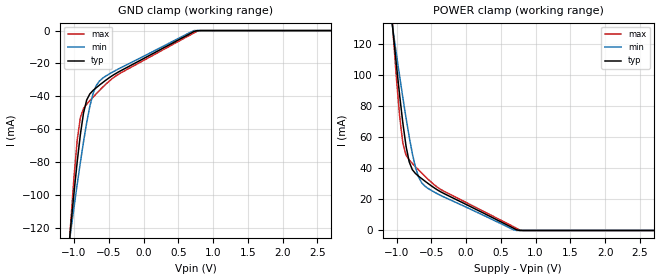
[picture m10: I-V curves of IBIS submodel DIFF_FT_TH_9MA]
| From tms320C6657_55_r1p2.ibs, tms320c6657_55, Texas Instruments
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|   Model Cell DIFF_FT_TH_9MA
|DIFF_FT_TH_9MA
[Submodel]   DIFF_FT_TH_9MA
Submodel_type   Dynamic_clamp
[POWER_clamp]
|   voltage   I(typ)   I(min)   I(max)
-1.5V     344.8mA    277.3mA    440.9mA
-1.091V   146.5mA    141.4mA    153.5mA
-1.046V   125.7mA    127mA      124.3mA
-954.6mV  86.42mA    98.78mA    72.95mA
-909.2mV  68.87mA    85.24mA    56mA
-863.7mV  54.18mA    72.3mA     48.37mA
-818.2mV  44.11mA    60.2mA     45.3mA
-727.3mV  36.59mA    40.46mA    40.96mA
-636.4mV  33.23mA    30.51mA    36.83mA
-545.5mV  30.15mA    26.97mA    32.86mA
772.8mV   0A         0A         343.5uA
3V        0A         0A         0A
[GND_clamp]
|   voltage   I(typ)   I(min)   I(max)
-1.5V     -337.5mA   -271.7mA   -431.5mA
-1.091V   -138.9mA   -136mA     -144.2mA
-1.046V   -118.3mA   -121.5mA   -115.4mA
-954.6mV  -79.8mA    -93.55mA   -66.73mA
-909.2mV  -63.2mA    -80.22mA   -52.89mA
-863.7mV  -50.14mA   -67.6mA    -47.4mA
-818.2mV  -42.21mA   -56.02mA   -44.78mA
-727.3mV  -36.46mA   -38.41mA   -40.54mA
-636.4mV  -33.23mA   -30.77mA   -36.5mA
-545.5mV  -30.26mA   -27.74mA   -32.71mA
772.8mV   0A         0A         -333.4uA
3V        0A         0A         0A
